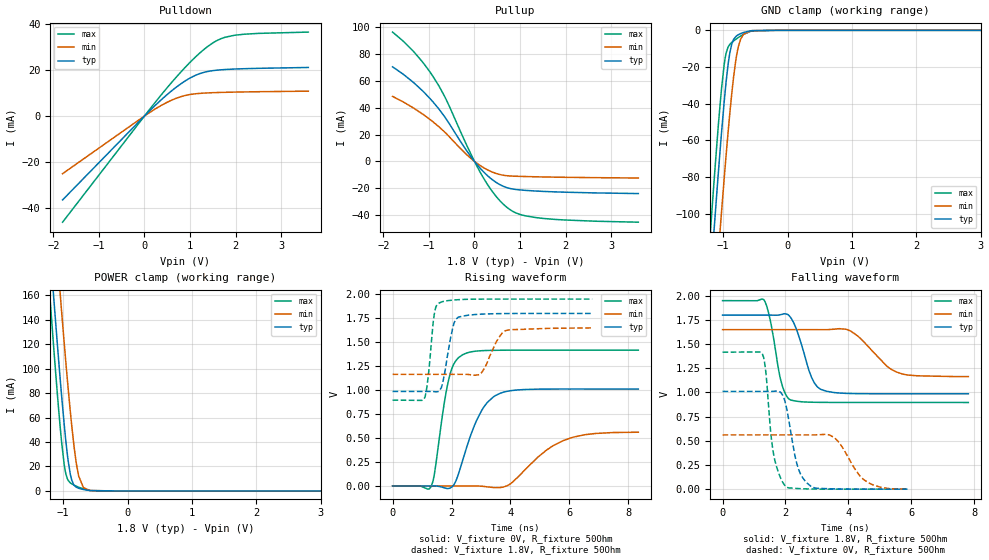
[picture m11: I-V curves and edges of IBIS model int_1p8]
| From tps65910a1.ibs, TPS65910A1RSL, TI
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|   int_1p8 Model
[Model]   int_1p8
Model_type   3-state
Polarity   Non-Inverting
Vmeas = 0.9
Vref = 0
Cref = 35pF
Rref = 100
|   typ   min   max
|   (nom PVT)   (fast PVT)   (slow PVT)
C_comp   8.728e-13   8.173e-13   1.047e-12
| Where nom  PVT is Nominal Process, 1.8V, 27C
|   Fast PVT is Strong Process,  1.95V, -40C
|   Slow PVT is Weak Process,   1.65V, 125C
[Voltage Range]   1.8   1.65   1.95
|Junction Temperature
[Temperature Range]   27   125   -40
[Pullup Reference]   1.8   1.65   1.95
[Pulldown Reference]   0   0   0
[Power Clamp Reference]   1.8   1.65   1.95
[GND Clamp Reference]   0   0   0
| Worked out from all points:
|   slope of the pulldown table from 0 to 0.27 V, typ, clamps not added: 51.7 ohm
|   slope of the pullup table from 0 to 0.27 V, typ, clamps not added: 26.7 ohm
|   GND clamp passes 1 mA (typ) near -0.66 V on its own axis
|   POWER clamp passes 1 mA (typ) near -0.67 V on its own axis
|   falling waveform, V_fixture 1.8V, R_fixture 50Ohm: 20-80 % time 473ps typ, 863ps min, 346ps max; typ from 1.8 V to 0.986 V
|   rising waveform, V_fixture 0V, R_fixture 50Ohm: 20-80 % time 751ps typ, 1.31ns min, 429ps max; typ from 0 V to 1.01 V
|   rising waveform, V_fixture 1.8V, R_fixture 50Ohm: 20-80 % time 286ps typ, 443ps min, 196ps max; typ from 0.986 V to 1.8 V
|   falling waveform, V_fixture 0V, R_fixture 50Ohm: 20-80 % time 368ps typ, 664ps min, 277ps max; typ from 1.01 V to 0 V
[Pulldown]
|   Voltage   I(typ)   I(min)   I(max)
-1.8V     -36.35mA   -24.99mA   -46mA
150uV     3.019uA    2.051uA    3.838uA
368.4mV   7.028mA    4.586mA    9.163mA
684mV     12.27mA    7.578mA    16.51mA
900mV     15.26mA    8.912mA    21.19mA
1.154V    17.9mA     9.686mA    26.18mA
1.381V    19.25mA    9.99mA     29.98mA
1.667V    19.98mA    10.2mA     33.37mA
1.98V     20.34mA    10.35mA    34.98mA
2.508V    20.64mA    10.51mA    35.78mA
3.6V      21.01mA    10.76mA    36.34mA
[GND Clamp]
|   Voltage   I(typ)   I(min)   I(max)
-1.8V     -448.9mA   -485.7mA   -427.4mA
-1.19V    -132.4mA   -176.2mA   -105.7mA
-1.147V   -111.5mA   -155.5mA   -84.81mA
-1.1V     -89.32mA   -133.3mA   -62.94mA
-1.046V   -64.82mA   -108.4mA   -39.78mA
-972mV    -34.5mA    -75.67mA   -15.8mA
-895.8mV  -12.11mA   -45.01mA   -7.602mA
-838mV    -4.983mA   -25.52mA   -5.782mA
-765.4mV  -2.427mA   -9.101mA   -3.964mA
-684.6mV  -1.171mA   -2.256mA   -2.222mA
-546.2mV  -149.7uA   -174.2uA   -341.2uA
3.6V      0A         0A         0A
[Pullup]
|   Voltage   I(typ)   I(min)   I(max)
-1.8V     70.38mA    48.38mA    96.23mA
-1.322V   58.19mA    39.35mA    81.18mA
-1.108V   51.39mA    34.46mA    72.51mA
-905.4mV  44.04mA    29.27mA    62.9mA
-620.2mV  31.47mA    20.65mA    45.91mA
-180mV    8.361mA    5.281mA    12.71mA
144mV     -5.787mA   -3.494mA   -9.198mA
467.8mV   -15.44mA   -8.889mA   -25.74mA
729.1mV   -19.7mA    -10.71mA   -34.63mA
1.006V    -21.23mA   -11.15mA   -39.54mA
1.474V    -22.26mA   -11.54mA   -42.3mA
3.6V      -23.93mA   -12.35mA   -45.23mA
[POWER Clamp]
|   Voltage   I(typ)   I(min)   I(max)
-1.8V     641.8mA    704.9mA    611.5mA
-1.225V   213.1mA    283.8mA    172.7mA
-1.195V   192.2mA    263mA      151.5mA
-1.147V   158.5mA    229.4mA    117.5mA
-1.043V   89.53mA    159.1mA    50.31mA
-983.2mV  54.16mA    120.9mA    21.49mA
-922.2mV  24.61mA    83.89mA    8.58mA
-867.6mV  9.027mA    53.96mA    5.819mA
-791.9mV  2.932mA    21.41mA    3.775mA
-684.6mV  1.138mA    2.656mA    1.614mA
-567.5mV  233.5uA    291.7uA    278.5uA
3.6V      0A         0A         0A
[Ramp]
R_load = 50
|   typ   min   max
dV/dt_r   0.606713/7.50902e-10   0.336836/1.30357e-09   0.850163/4.28303e-10
dV/dt_f   0.488157/4.71529e-10   0.291143/8.57505e-10   0.632001/3.43973e-10
[Falling Waveform]
V_fixture = 1.8V
V_fixture_min = 1.65V
V_fixture_max = 1.95V
R_fixture = 50Ohm
|   Time   V(typ)   V(min)   V(max)
0s        1.8V       1.65V      1.95V
1.322ns   1.8V       1.65V      1.955V
1.518ns   1.8V       1.65V      1.745V
1.844ns   1.805V     1.65V      1.135V
2.162ns   1.777V     1.65V      922.6mV
2.83ns    1.155V     1.65V      899.3mV
3.116ns   1.033V     1.65V      898mV
4.088ns   989.3mV    1.632V     896.9mV
5.732ns   986.5mV    1.19V      896.9mV
7.812ns   986.4mV    1.165V     896.7mV
[Rising Waveform]
V_fixture = 0V
V_fixture_min = 0V
V_fixture_max = 0V
R_fixture = 50Ohm
|   Time   V(typ)   V(min)   V(max)
0s        366.7pV    827.3pV    342.3pV
1.308ns   252.6uV    -19.01nV   -4.573mV
1.416ns   945.4uV    11.02nV    119.4mV
1.908ns   -25.75mV   1.268uV    1.115V
2.132ns   41.88mV    -3.541uV   1.3V
2.378ns   267.6mV    -28.97uV   1.37V
3.032ns   793mV      -2.719mV   1.412V
3.664ns   968.8mV    -15.77mV   1.416V
5.796ns   1.011V     474.5mV    1.417V
8.336ns   1.011V     561mV      1.417V
[Rising Waveform]
V_fixture = 1.8V
V_fixture_min = 1.65V
V_fixture_max = 1.95V
R_fixture = 50Ohm
|   Time   V(typ)   V(min)   V(max)
0s        986.1mV    1.165V     895.5mV
1.076ns   986.1mV    1.165V     912.3mV
1.202ns   986.1mV    1.165V     1.124V
1.406ns   984.2mV    1.165V     1.775V
1.582ns   991.8mV    1.165V     1.909V
2.074ns   1.688V     1.165V     1.94V
2.236ns   1.762V     1.165V     1.944V
2.958ns   1.792V     1.165V     1.949V
3.872ns   1.799V     1.624V     1.95V
6.77ns    1.8V       1.649V     1.95V
[Falling Waveform]
V_fixture = 0V
V_fixture_min = 0V
V_fixture_max = 0V
R_fixture = 50Ohm
|   Time   V(typ)   V(min)   V(max)
0s        1.011V     561.4mV    1.417V
1.266ns   1.011V     561.4mV    1.397V
1.374ns   1.011V     561.4mV    1.215V
1.636ns   1.012V     561.4mV    336.8mV
2.034ns   838.7mV    561.4mV    22.84mV
2.362ns   262.1mV    561.4mV    7.204mV
2.818ns   27.29mV    561.2mV    1.668mV
3.572ns   2.886mV    529mV      128.9uV
4.634ns   140.2uV    67.34mV    42.24uV
5.88ns    22.05uV    138.2uV    18.88uV
